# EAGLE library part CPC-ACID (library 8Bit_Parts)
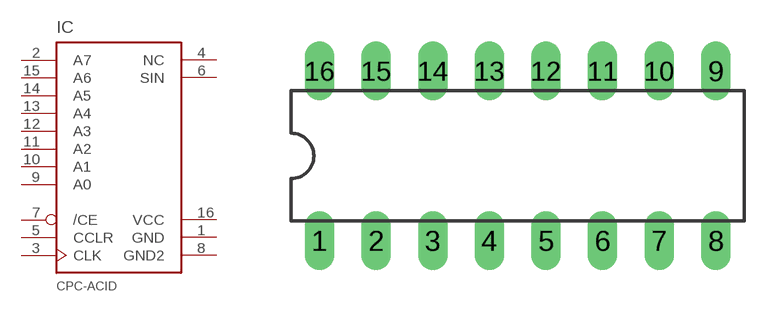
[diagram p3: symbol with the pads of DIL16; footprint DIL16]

Designator prefix IC

## CPC-ACID  [DIL16]
1  GND  pwr
2  A7  in
3  CLK  in
4  NC  nc
5  CCLR  in
6  SIN  out
7  /CE  in
8  GND2  pwr
9  A0  in
10  A1  in
11  A2  in
12  A3  in
13  A4  in
14  A5  in
15  A6  in
16  VCC  pwr

## Footprint DIL16 (pad centres in mm)
Dual In Line Package
drill 0.813 long: 1 -8.89,-3.81; 2 -6.35,-3.81; 3 -3.81,-3.81; 4 -1.27,-3.81; 5 1.27,-3.81; 6 3.81,-3.81; 7 6.35,-3.81; 8 8.89,-3.81; 9 8.89,3.81; 10 6.35,3.81; 11 3.81,3.81; 12 1.27,3.81; 13 -1.27,3.81; 14 -3.81,3.81; 15 -6.35,3.81; 16 -8.89,3.81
